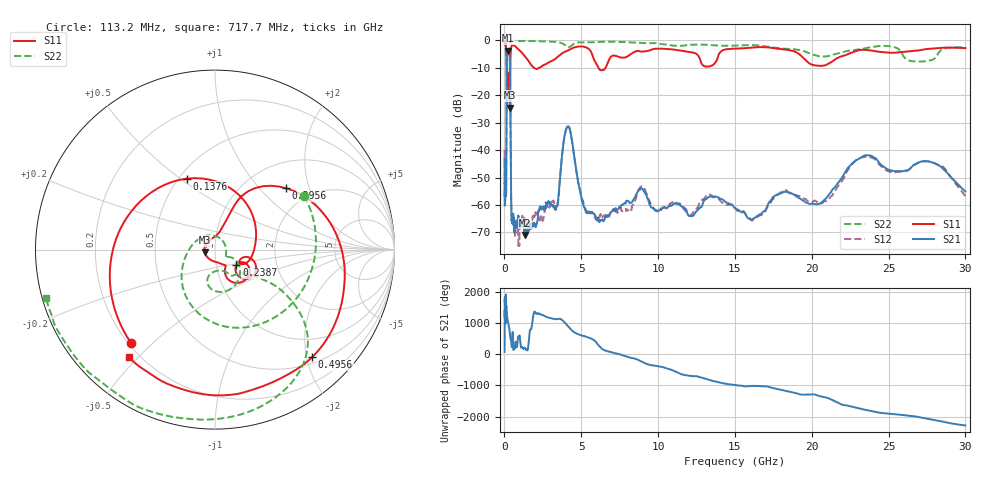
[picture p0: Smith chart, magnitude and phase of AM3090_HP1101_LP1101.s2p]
! Date/Time: Thu, Feb 28, 2019 2:08 PM
! Network Analyzer: Agilent Technologies E8364B Rev: A.07.50.67
! Sweep from 0.010 to 30.000 GHz, 1601 Points, Sweep Type: LOG
! Power Supply: 5.022 V, 0.002 A
# Hz S DB R 50
!freq MagS11 AngS11 MagS21 AngS21 MagS12 AngS12 MagS22 AngS22
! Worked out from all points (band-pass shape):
!   1601 points, 10 MHz to 30 GHz, reference 50 ohm
!   highest |S21| = -3.83 dB at 243.5 MHz (marker M1); lowest = -70.9 dB at 1.328 GHz (marker M2)
!   |S21| within 3 dB of the highest: 154.2 MHz to 348.3 MHz (194.1 MHz wide, 77.3 % of centre)
!   lowest |S11| = -24.5 dB at 343.9 MHz (marker M3), VSWR 1.13, Z = 44.6 - j1.44 ohm
!   |S11| at or under -10 dB: 144.1 MHz to 382.9 MHz (238.8 MHz wide, 90.6 % of centre); 1.9 GHz to 2.267 GHz (366.8 MHz wide, 17.6 % of centre); 6.111 GHz to 6.584 GHz (472.7 MHz wide, 7.45 % of centre)
!   |S22| runs from -24.3 to -0.1 dB; largest |S21 - S12| = 0.014
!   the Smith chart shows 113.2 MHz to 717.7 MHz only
!   S11 on the Smith chart (normalised r, x): 113.2 MHz: 0.21, -0.43; 137.6 MHz: 0.55, +0.53; 238.7 MHz: 1.25, -0.22; 395.6 MHz: 1.50, +1.42; 495.6 MHz: 0.61, -2.11; 717.7 MHz: 0.16, -0.47
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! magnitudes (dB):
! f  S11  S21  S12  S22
! 10 MHz  -0.2  -42.9  -40.0  -0.7
! 38.04 MHz  -0.4  -57.2  -56.9  -1.5
! 113.2 MHz  -3.1  -54.4  -53.6  -4.7
! 137.6 MHz  -7.4  -20.5  -20.5  -8.7
! 144.7 MHz  -10.3  -11.8  -11.7  -17.5
! 238.7 MHz  -16.6  -3.8  -3.8  -16.1
! 243.5 MHz  -16.5  -3.8  -3.8  -16.9
! 343.9 MHz  -24.5  -6.4  -6.4  -11.8
! 395.6 MHz  -5.6  -31.6  -31.7  -1.5
! 439.5 MHz  -2.6  -58.3  -59.0  -0.5
! 495.6 MHz  -1.9  -65.6  -64.4  -0.2
! 550.5 MHz  -1.9  -63.6  -64.7  -0.2
! 717.7 MHz  -2.3  -67.0  -69.7  -0.2
! 1.328 GHz  -5.8  -70.9  -65.7  -0.3
! 2.084 GHz  -10.5  -67.0  -63.0  -0.4
! 3.385 GHz  -6.4  -60.8  -61.2  -0.7
! 4.115 GHz  -3.8  -31.4  -31.4  -2.5
! 5.285 GHz  -2.6  -62.2  -61.7  -0.8
! 7.926 GHz  -6.1  -58.5  -62.2  -0.7
! 16.29 GHz  -2.6  -64.5  -65.1  -1.8
! 23.48 GHz  -3.5  -41.9  -42.4  -3.0
! 30 GHz  -2.9  -55.1  -56.8  -2.5
